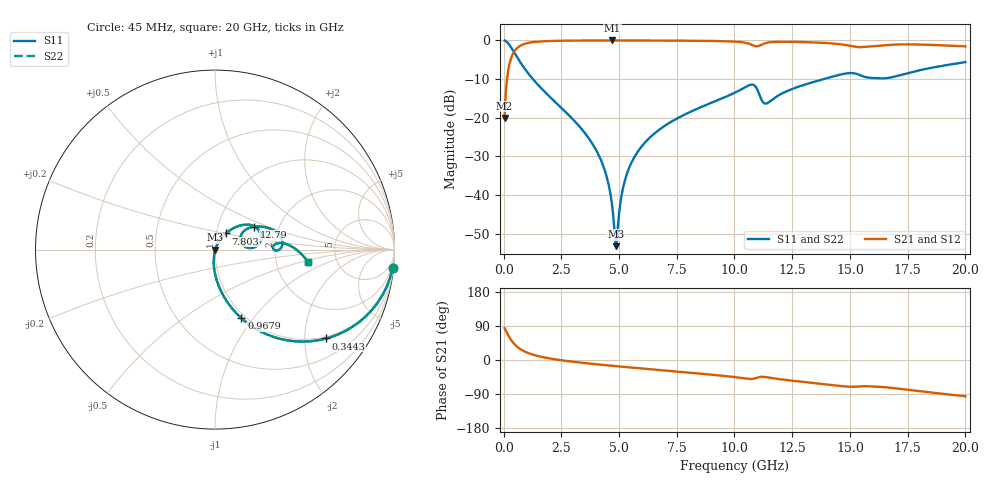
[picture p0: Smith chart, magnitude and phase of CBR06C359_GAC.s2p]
! S-parameter model data by Modelithics Inc.  support@modelithics.com 813-866-6335  Tampa FL USA
! S-Parameter data specifications:
! Substrate: 20-mil Rogers 4350B, substrate thickness, H=0.508mm, Dielectric constant, Er=3.75
! PCB Mounting Pad Footprint: Pad width, PadW=0.85mm , Pad length, PadL=0.64mm , Pad gap, PadG (edge-to-edge)=0.62mm , Reference planes=1.9mm apart
#  GHz  S  MA  R 50
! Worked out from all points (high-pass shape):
!   801 points, 45 MHz to 20 GHz, reference 50 ohm
!   highest |S21| = -0.02 dB at 4.709 GHz (marker M1); lowest = -20.1 dB at 45 MHz (marker M2)
!   |S21| within 3 dB of the highest: 447.4 MHz to end of sweep
!   lowest |S11| = -53.3 dB at 4.859 GHz (marker M3), VSWR 1.00, Z = 50.2 - j0.102 ohm
!   |S11| at or under -10 dB: 1.267 GHz to 13.87 GHz (12.6 GHz wide, 167 % of centre)
!   |S22| runs from -53.3 to 0.0 dB; largest |S21 - S12| = 0
!   S11 on the Smith chart (normalised r, x): 45 MHz: 1, -20; 344.3 MHz: 0.95, -2.54; 967.9 MHz: 0.95, -0.87; 7.803 GHz: 1.11, +0.20; 12.79 GHz: 1.49, +0.41; 20 GHz: 3.07, -0.58
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0.045  0.9951 -5.8  0.09921 84.2  0.09921 84.2  0.9951 -5.8
0.194662  0.9179 -24.0  0.3964 66.0  0.3964 66.0  0.9179 -24.0
0.344325  0.7935 -38.6  0.6081 51.4  0.6081 51.4  0.7935 -38.6
0.618706  0.5832 -56.3  0.8116 33.6  0.8116 33.6  0.5832 -56.3
0.967919  0.4093 -68.9  0.9114 20.9  0.9114 20.9  0.4093 -68.9
3.387462  0.07079 -95.8  0.9955 -7.3  0.9955 -7.3  0.07079 -95.8
4.285437  0.02507 -98.3  0.9975 -12.9  0.9975 -12.9  0.02507 -98.3
4.534875  0.01415 -96.0  0.9976 -14.3  0.9976 -14.3  0.01415 -96.0
4.709481  0.006932 -87.8  0.9976 -15.3  0.9976 -15.3  0.006932 -87.8
4.859144  0.002169 -28.1  0.9976 -16.2  0.9976 -16.2  0.002169 -28.1
5.158469  0.0117 61.3  0.9975 -17.9  0.9975 -17.9  0.0117 61.3
5.457794  0.02311 64.8  0.9972 -19.5  0.9972 -19.5  0.02311 64.8
6.704981  0.06847 61.5  0.9946 -26.2  0.9946 -26.2  0.06847 61.5
7.802506  0.1081 56.2  0.9905 -32.1  0.9905 -32.1  0.1081 56.2
10.0225  0.2108 41.0  0.9633 -45.2  0.9633 -45.2  0.2108 41.0
10.79576  0.2676 17.4  0.8651 -49.9  0.8651 -49.9  0.2676 17.4
11.36946  0.152 19.4  0.925 -45.3  0.925 -45.3  0.152 19.4
12.79126  0.2526 30.2  0.9528 -56.6  0.9528 -56.6  0.2526 30.2
13.36496  0.2861 26.6  0.9424 -60.4  0.9424 -60.4  0.2861 26.6
14.96136  0.3772 8.2  0.8544 -70.5  0.8544 -70.5  0.3772 8.2
16.68248  0.3274 4.0  0.8719 -72.7  0.8719 -72.7  0.3274 4.0
20  0.5226 -7.5  0.8357 -95.8  0.8357 -95.8  0.5226 -7.5
